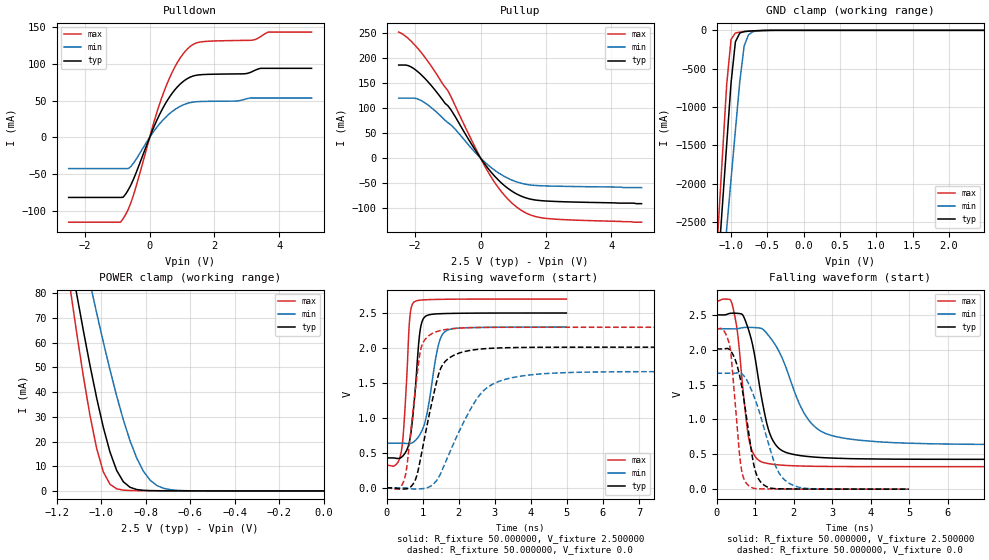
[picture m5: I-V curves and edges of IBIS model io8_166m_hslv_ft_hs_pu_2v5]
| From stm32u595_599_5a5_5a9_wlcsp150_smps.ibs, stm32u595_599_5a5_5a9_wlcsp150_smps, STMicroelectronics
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|   Model io8_166m_hslv_ft_hs_pu_2v5
[Model]  io8_166m_hslv_ft_hs_pu_2v5
Model_type I/O
Polarity   Non-Inverting
Enable   Active-Low
Vinl =   0.750000V
Vinh =   1.750000V
Vmeas =  1.250000V
Cref =   50.000000pF
Rref =   100.000000M
Vref =   0.0V
C_comp   3.458600pF   3.458000pF   3.495600pF
[Temperature Range]   25.000000   0.140000k   -40.000000
[Pullup Reference]   2.500000V   2.300000V   2.700000V
[Pulldown Reference]   0.0V   0.0V   0.0V
[POWER Clamp Reference]   2.500000V   2.300000V   2.700000V
[GND Clamp Reference]   0.0V   0.0V   0.0V
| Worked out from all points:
|   slope of the pulldown table from 0 to 0.375 V, typ, clamps not added: 10.1 ohm
|   slope of the pullup table from 0 to 0.375 V, typ, clamps not added: 11.7 ohm
|   GND clamp passes 1 mA (typ) near -0.50 V on its own axis
|   POWER clamp passes 1 mA (typ) near -0.85 V on its own axis
|   rising waveform, R_fixture 50.000000, V_fixture 2.500000: 20-80 % time 205ps typ, 325ps min, 149ps max; typ from 0.428 V to 2.5 V
|   rising waveform, R_fixture 50.000000, V_fixture 0.0: 20-80 % time 499ps typ, 980ps min, 303ps max; typ from 0 V to 2.01 V
|   falling waveform, R_fixture 50.000000, V_fixture 2.500000: 20-80 % time 425ps typ, 792ps min, 267ps max; typ from 2.5 V to 0.428 V
|   falling waveform, R_fixture 50.000000, V_fixture 0.0: 20-80 % time 342ps typ, 563ps min, 213ps max; typ from 2.01 V to 0 V
[Pulldown]
|Voltage   I(typ)   I(min)   I(max)
-2.5V     -81.62mA   -42.31mA   -115.3mA
-900mV    -81.62mA   -42.31mA   -115.3mA
-820mV    -81.43mA   -42.31mA   -110.6mA
-500mV    -56.95mA   -35.08mA   -78.57mA
140mV     15.18mA    9.02mA     22.02mA
460mV     44mA       25.98mA    64.38mA
860mV     68.91mA    40.27mA    102.2mA
1.26V     82.21mA    47.42mA    124mA
1.66V     85.54mA    49mA       130.3mA
3.18V     89.84mA    53.62mA    132.3mA
3.66V     93.97mA    53.62mA    143.3mA
5V        93.97mA    53.62mA    143.3mA
[Pullup]
|Voltage   I(typ)   I(min)   I(max)
-2.5V     185.5mA    119.5mA    251.2mA
-2.12V    181.7mA    119.5mA    233.1mA
-1.88V    170.2mA    116.8mA    215.9mA
-1.64V    154.6mA    107.5mA    195.7mA
-1V       104.5mA    70.67mA    134.6mA
-120mV    11.81mA    8.047mA    15.6mA
280mV     -24.74mA   -16.62mA   -33.17mA
680mV     -52.22mA   -34.93mA   -70.46mA
1.08V     -70.88mA   -47.09mA   -96.6mA
1.48V     -81.29mA   -53.4mA    -112.4mA
1.96V     -85.56mA   -55.61mA   -120.1mA
4.92V     -91mA      -59mA      -128mA
[GND_clamp]
|Voltage   I(typ)   I(min)   I(max)
-2.5V     -9.641A    -9.693A    -9.352A
-1.18V    -3.114A    -3.874A    -2.614A
-1.12V    -2.301A    -3.23A     -1.656A
-1.06V    -1.489A    -2.587A    -706.2mA
-1V       -685.8mA   -1.945A    -119.3mA
-940mV    -149.7mA   -1.304A    -34.73mA
-880mV    -35.54mA   -672.6mA   -23.06mA
-820mV    -16.2mA    -206.4mA   -17.27mA
-760mV    -10.58mA   -57.55mA   -12.41mA
-700mV    -7.152mA   -18.74mA   -8.24mA
-400mV    -103.3uA   -378.6uA   -41.75uA
2.48V     0A         13.22nA    0A
[POWER_clamp]
|Voltage   I(typ)   I(min)   I(max)
-2.49V    881.1mA    773.1mA    1.07A
-1.14V    95.32mA    122.8mA    82.93mA
-1.11V    79.97mA    109.7mA    64.26mA
-1.05V    50.95mA    84.3mA     30.69mA
-1.02V    37.7mA     72.08mA    17.29mA
-990mV    25.79mA    60.29mA    7.738mA
-930mV    8.312mA    38.47mA    853.1uA
-900mV    3.712mA    28.81mA    313.6uA
-840mV    566.2uA    13.29mA    123.7uA
-780mV    119uA      4.365mA    94.04uA
-660mV    38.98uA    251.5uA    57.76uA
0V        0A         18.93nA    0A
[Ramp]
| variable   typ   min   max
dV/dt_r  1.20644/0.49873n   0.99753/0.97806n   1.37763/0.30223n
dV/dt_f  1.24313/0.42470n   0.99677/0.79016n   1.42607/0.26629n
R_load = 50.000000
[Rising Waveform]
R_fixture= 50.000000
V_fixture= 2.500000
V_fixture_min= 2.300000
V_fixture_max= 2.700000
|time   V(typ)   V(min)   V(max)
0s        428.1mV    638.2mV    323.2mV
410.4ps   436.2mV    638.3mV    522.7mV
500.5ps   487.2mV    636.9mV    1.039V
640.6ps   675.7mV    633.5mV    2.408V
750.8ps   1.138V     656.1mV    2.652V
900.9ps   2.116V     742.4mV    2.681V
981ps     2.37V      817.9mV    2.686V
1.431ns   2.488V     2.027V     2.695V
1.642ns   2.492V     2.242V     2.696V
4.985ns   2.5V       2.3V       2.699V
[Rising Waveform]
R_fixture= 50.000000
V_fixture= 0.0
V_fixture_min= 0.0
V_fixture_max= 0.0
|time   V(typ)   V(min)   V(max)
0s        419.5uV    535.6uV    411.3uV
500.5ps   -16.14mV   -161.3uV   132.6mV
780.8ps   96.43mV    -16.69mV   1.323V
940.9ps   413.7mV    -13.67mV   1.964V
1.301ns   1.325V     54.8mV     2.216V
1.502ns   1.708V     207.8mV    2.25V
1.762ns   1.865V     519.3mV    2.273V
2.503ns   1.979V     1.272V     2.292V
3.163ns   2.002V     1.531V     2.295V
9.97ns    2.011V     1.663V     2.296V
[Falling Waveform]
R_fixture= 50.000000
V_fixture= 2.500000
V_fixture_min= 2.300000
V_fixture_max= 2.700000
|time   V(typ)   V(min)   V(max)
0s        2.5V       2.3V       2.699V
400.4ps   2.524V     2.3V       2.662V
540.5ps   2.522V     2.301V     2.259V
840.8ps   2.268V     2.321V     713.6mV
1.161ns   1.333V     2.306V     393.1mV
1.361ns   829.2mV    2.195V     365.5mV
1.622ns   583.4mV    1.976V     347.9mV
2.262ns   475.4mV    1.098V     331.3mV
2.843ns   450mV      795.5mV    326.5mV
9.97ns    428.1mV    638.2mV    323.2mV
[Falling Waveform]
R_fixture= 50.000000
V_fixture= 0.0
V_fixture_min= 0.0
V_fixture_max= 0.0
|time   V(typ)   V(min)   V(max)
0s        2.011V     1.663V     2.296V
180.2ps   2.011V     1.663V     2.279V
340.3ps   2V         1.663V     2.061V
620.6ps   1.569V     1.664V     380.1mV
820.8ps   862.5mV    1.527V     56.56mV
971ps     337.3mV    1.329V     12.74mV
1.111ns   127.7mV    1.106V     5.796mV
1.542ns   7.231mV    320.6mV    2.685mV
1.872ns   3.967mV    88.11mV    1.751mV
4.985ns   419.5uV    535.6uV    411.3uV
